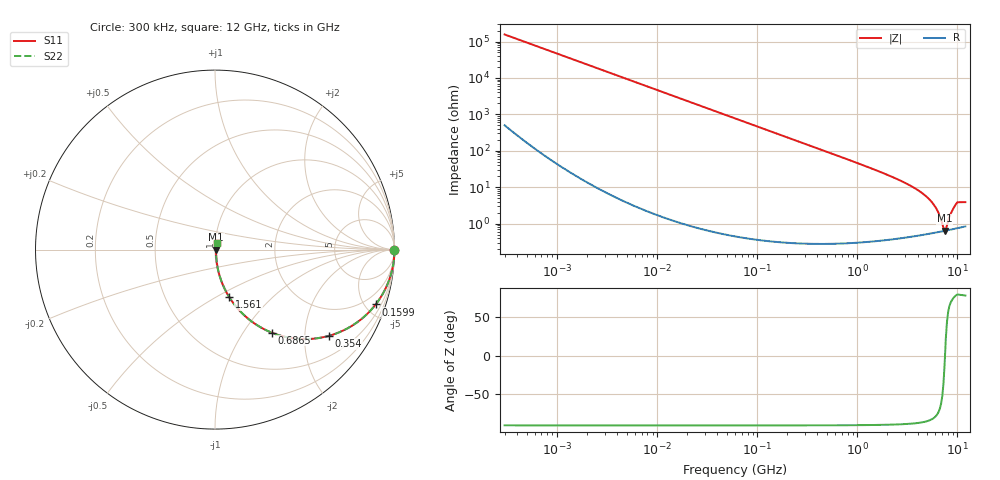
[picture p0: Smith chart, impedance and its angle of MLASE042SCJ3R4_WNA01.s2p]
! MLASE042SCJ3R4_WNA01  S-PARAMETER MODEL  ( General Type )
! Model Generated by TAIYO YUDEN Corporation (http://www.ty-top.com)
! Version 1.0
! TAIYO YUDEN Control No. 120810
! Copyright(c) 2012 TAIYO YUDEN CO.,LTD. All Rights Reserved.
! Product Description (link to TY-COMPAS)
! https://ds.yuden.co.jp/TYCOMPAS/or/detail?pn=MLASE042SCJ3R4BWNA01&u=M
! Products Name : Multilayer Ceramic Capacitors
! Characteristics :
!  Capacitance : 3.4 pF , Rated Voltage : 16V , TCC : CJ / C0J
!  Case Size : 0.4 x 0.2 / 0.016 x 0.008 [mm/inch] , Thickness : 0.2 / 0.008 [mm/inch]
!  (Conditions: Temperature = 25 degC , DC Bias Current/Voltage = 0A / 0V)
! External Node Assignments :
!  1  o---| |---o  2
! GND o---------o GND
! Frequency Range : 0.3MHz  -  12000MHz  [ 401 STEP ]
# MHz S RI R 50
! Freq[MHz].  S11 Real  S11 Imag  S21 Real  S21 Imag  S12 Real  S12 Imag  S22 Real  S22 Imag
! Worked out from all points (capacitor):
!   401 points, 300 kHz to 12 GHz, reference 50 ohm
!   read as one part in series: C = 3.4 pF near 316.3 kHz
!   lowest |Z| = 642 mohm at 7.449 GHz (marker M1)
!   series resonance near 7.508 GHz, so ESL is about 130 pH
!   S11 on the Smith chart (normalised r, x): 300 kHz: open; 159.9 MHz: 1.01, -5.86; 354 MHz: 1.01, -2.64; 686.5 MHz: 1.01, -1.35; 1.561 GHz: 1.01, -0.57; 12 GHz: 1.02, +0.08
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0.3  1 -0.00064  2.46e-06 0.00064  2.46e-06 0.00064  1 -0.00064
1.769972  1 -0.00378  1.66e-05 0.00378  1.66e-05 0.00378  1 -0.00378
10.44266  0.9995 -0.0223  0.000505 0.0223  0.000505 0.0223  0.9995 -0.0223
60  0.9838 -0.126  0.0162 0.126  0.0162 0.126  0.9838 -0.126
159.8975  0.8954 -0.3056  0.1046 0.3056  0.1046 0.3056  0.8954 -0.3056
237.9135  0.7944 -0.4034  0.2056 0.4034  0.2056 0.4034  0.7944 -0.4034
353.9943  0.6353 -0.4803  0.3647 0.4803  0.3647 0.4803  0.6353 -0.4803
686.4755  0.3149 -0.4624  0.6851 0.4624  0.6851 0.4624  0.3149 -0.4624
1021.415  0.1702 -0.3725  0.8298 0.3725  0.8298 0.3725  0.1702 -0.3725
1560.575  0.0788 -0.2638  0.9212 0.2638  0.9212 0.2638  0.0788 -0.2638
2088.533  0.0443 -0.1972  0.9557 0.1972  0.9557 0.1972  0.0443 -0.1972
3547.679  0.0147 -0.1007  0.9853 0.1007  0.9853 0.1007  0.0147 -0.1007
5006.236  0.00778 -0.0514  0.9922 0.0514  0.9922 0.0514  0.00778 -0.0514
5565.855  0.00681 -0.0376  0.9932 0.0376  0.9932 0.0376  0.00681 -0.0376
6188.031  0.00628 -0.0241  0.9937 0.0241  0.9937 0.0241  0.00628 -0.0241
7064.448  0.00616 -0.00764  0.9938 0.00764  0.9938 0.00764  0.00616 -0.00764
7448.838  0.00628 -0.00109  0.9937 0.00109  0.9937 0.00109  0.00628 -0.00109
7854.144  0.0065 0.00604  0.9935 -0.00604  0.9935 -0.00604  0.0065 0.00604
8732.115  0.00725 0.0195  0.9928 -0.0195  0.9928 -0.0195  0.00725 0.0195
9708.23  0.00844 0.0336  0.9916 -0.0336  0.9916 -0.0336  0.00844 0.0336
10511.28  0.00906 0.0373  0.9909 -0.0373  0.9909 -0.0373  0.00906 0.0373
12000  0.0097 0.0373  0.9903 -0.0373  0.9903 -0.0373  0.0097 0.0373
